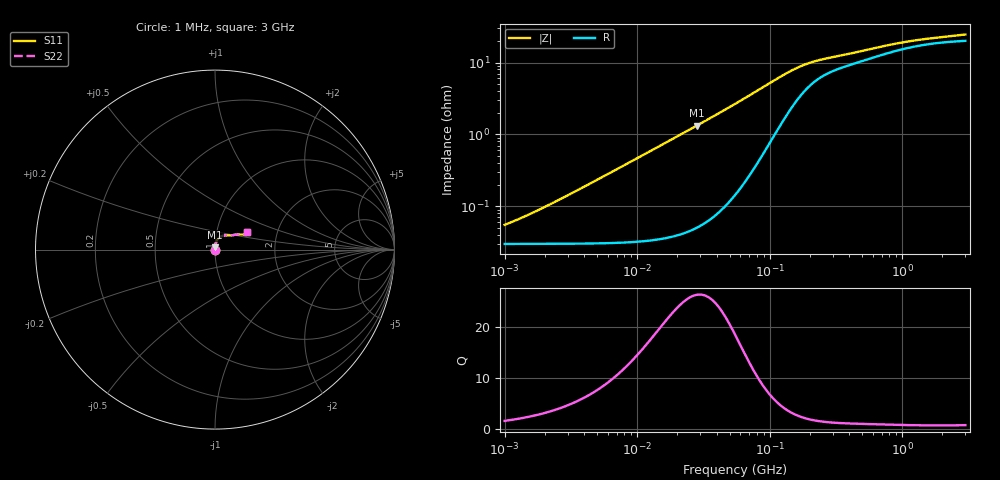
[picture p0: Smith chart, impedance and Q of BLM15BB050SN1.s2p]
! BLM15BB050SN1
# Hz S RI R 50
!Freq.(Hz) S11(Real) S11(Imag) S21(Real) S21(Imag) S12(Real) S12(Imag) S22(Real) S22(Imag)
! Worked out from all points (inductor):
!   401 points, 1 MHz to 3 GHz, reference 50 ohm
!   read as one part in series: L = 7.39 nH near 1.975 MHz
!   highest Q = 26.3 at 28.29 MHz (marker M1), where L = 7.48 nH
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1000000  0.0003 0.000464  0.9997 -0.000464  0.9997 -0.000464  0.0003 0.000464
1040844  0.0003 0.000483  0.9997 -0.000483  0.9997 -0.000483  0.0003 0.000483
1221597  0.000301 0.000567  0.9997 -0.000567  0.9997 -0.000567  0.000301 0.000567
1716745  0.000301 0.000797  0.9997 -0.000797  0.9997 -0.000797  0.000301 0.000797
2461366  0.000303 0.00114  0.9997 -0.00114  0.9997 -0.00114  0.000303 0.00114
3823119  0.000306 0.00177  0.9997 -0.00177  0.9997 -0.00177  0.000306 0.00177
1.461624e7  0.000394 0.00681  0.9996 -0.00681  0.9996 -0.00681  0.000394 0.00681
2.829425e7  0.000681 0.0133  0.9993 -0.0133  0.9993 -0.0133  0.000681 0.0133
5.477226e7  0.00213 0.0264  0.9979 -0.0264  0.9979 -0.0264  0.00213 0.0264
9.216659e7  0.008 0.0461  0.992 -0.0461  0.992 -0.0461  0.008 0.0461
1.148668e8  0.0148 0.0576  0.9852 -0.0576  0.9852 -0.0576  0.0148 0.0576
1.348146e8  0.0228 0.0661  0.9772 -0.0661  0.9772 -0.0661  0.0228 0.0661
1.680187e8  0.038 0.0753  0.962 -0.0753  0.962 -0.0753  0.038 0.0753
1.857042e8  0.0458 0.0777  0.9542 -0.0777  0.9542 -0.0777  0.0458 0.0777
2.094008e8  0.055 0.0791  0.945 -0.0791  0.945 -0.0791  0.055 0.0791
2.558035e8  0.0685 0.079  0.9315 -0.079  0.9315 -0.079  0.0685 0.079
4.0536e8  0.0918 0.0794  0.9082 -0.0794  0.9082 -0.0794  0.0918 0.0794
8.005644e8  0.1286 0.0845  0.8714 -0.0845  0.8714 -0.0845  0.1286 0.0845
1.017911e9  0.1417 0.0844  0.8583 -0.0844  0.8583 -0.0844  0.1417 0.0844
1.320433e9  0.1539 0.0838  0.8461 -0.0838  0.8461 -0.0838  0.1539 0.0838
2.050964e9  0.1689 0.0864  0.8311 -0.0864  0.8311 -0.0864  0.1689 0.0864
3e9  0.1783 0.0973  0.8217 -0.0973  0.8217 -0.0973  0.1783 0.0973
